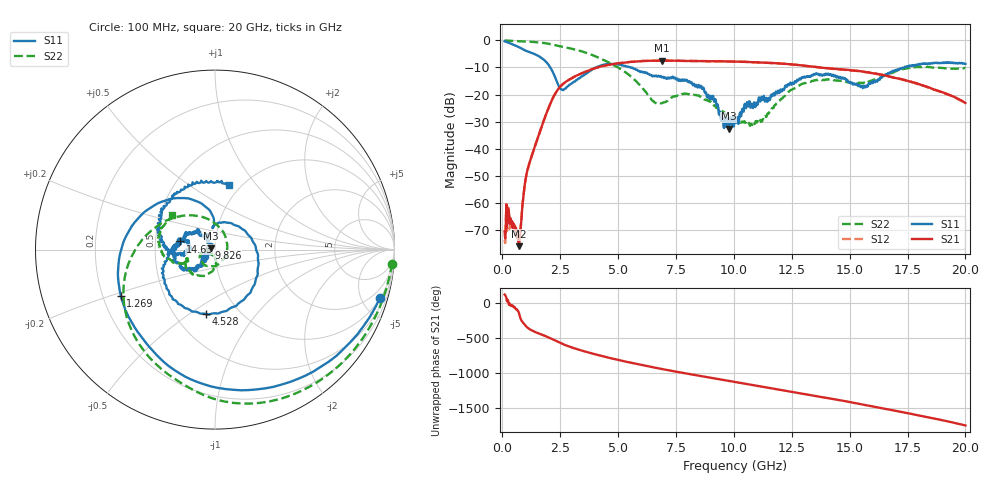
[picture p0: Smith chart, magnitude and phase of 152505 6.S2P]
!  2-Port S-parameters saved by WinCal
! VAR MeasName=S-Parameters (CALIBRATED_DATA) read from VNA (N5230C)
! VAR MeasDate=4/10/2015 9:28:59 AM
! VAR NAME=152505 6
! VAR FILENAME=152505 6.S2P
! VAR DATE=4/10/2015 9:28:59 AM
! VAR PHYS_PORTS=1,2
# Hz S DB R 50
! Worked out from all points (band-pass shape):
!   801 points, 100 MHz to 20 GHz, reference 50 ohm
!   highest |S21| = -7.48 dB at 6.891 GHz (marker M1); lowest = -75.8 dB at 721.9 MHz (marker M2)
!   |S21| within 3 dB of the highest: 3.941 GHz to 14.26 GHz (10.32 GHz wide, 113 % of centre)
!   lowest |S11| = -32.6 dB at 9.776 GHz (marker M3), VSWR 1.05, Z = 47.8 + j0.646 ohm
!   |S11| at or under -10 dB: 2.075 GHz to 4.059 GHz (1.984 GHz wide, 64.7 % of centre); 5.532 GHz to 17.36 GHz (11.83 GHz wide, 103 % of centre)
!   |S22| runs from -31.5 to -0.1 dB; largest |S21 - S12| = 0.0059
!   S11 on the Smith chart (normalised r, x): 100 MHz: 1.03, -6.80; 1.269 GHz: 0.28, -0.22; 4.528 GHz: 0.71, -0.58; 9.826 GHz: 0.93, +0.02; 14.63 GHz: 0.67, +0.06; 20 GHz: 0.89, +0.73
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1e8  -0.37 -16.4  -70.50 126.7  -73.55 148.1  -0.08 -4.6
2.4925e8  -0.86 -37.6  -62.04 42.8  -61.55 44.8  -0.17 -10.6
7.21875e8  -2.56 -97.3  -75.81 -140.8  -74.99 -134.5  -0.34 -29.3
1.020375e9  -3.89 -129.0  -50.46 36.0  -50.54 36.4  -0.46 -41.3
1.269125e9  -4.66 -153.9  -42.65 -25.8  -42.61 -25.6  -0.59 -51.4
1.965625e9  -8.67 129.3  -25.58 -121.0  -25.63 -121.1  -1.24 -81.0
2.5875e9  -18.20 96.5  -16.34 143.1  -16.38 143.1  -2.41 -106.5
3.43325e9  -13.38 13.5  -12.16 45.7  -12.14 46.0  -4.10 -141.5
4.52775e9  -8.84 -97.9  -9.16 -50.8  -9.14 -50.7  -7.87 171.1
5.448125e9  -9.86 -153.4  -8.07 -120.1  -8.03 -120.1  -12.63 125.2
6.741625e9  -13.05 174.4  -7.52 152.3  -7.48 151.9  -23.46 -10.3
6.890875e9  -13.71 175.1  -7.48 142.8  -7.50 142.6  -23.16 -34.5
8.10975e9  -15.55 148.9  -7.63 69.2  -7.67 68.9  -20.02 -136.0
9.776375e9  -32.60 163.2  -7.81 -26.7  -7.83 -26.8  -28.01 -169.1
9.826125e9  -28.64 163.9  -7.81 -29.7  -7.79 -29.8  -28.57 -164.5
1.005e10  -27.71 -151.5  -7.85 -42.8  -7.86 -42.9  -29.71 -157.6
1.119425e10  -20.84 -140.2  -8.21 -108.4  -8.19 -108.8  -29.99 -100.7
1.196538e10  -19.46 -129.7  -8.55 -153.0  -8.56 -152.9  -22.14 -86.0
1.338325e10  -12.95 -160.2  -9.72 124.9  -9.66 125.0  -14.96 -125.8
1.4627e10  -14.07 166.6  -10.72 54.1  -10.77 53.6  -14.94 -159.4
1.669162e10  -12.21 -175.0  -13.29 -75.6  -13.32 -76.6  -12.34 -162.2
2e10  -8.70 77.6  -23.10 55.9  -23.11 56.6  -10.21 141.5
